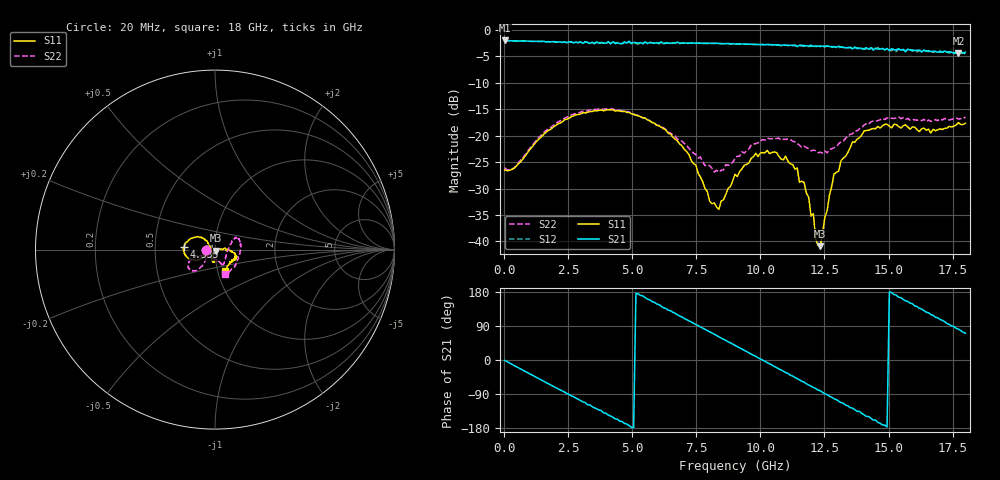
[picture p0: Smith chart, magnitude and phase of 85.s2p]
!Agilent Technologies,N5230A,US43500223,A.07.50.48
!Agilent N5230A: A.07.50.48
!Date: Monday, January 11, 2016 20:00:36
!Correction: S11(Full 2 Port(1,2))
!S21(Full 2 Port(1,2))
!S12(Full 2 Port(1,2))
!S22(Full 2 Port(1,2))
!S2P File: Measurements: S11, S21, S12, S22:
# Hz S  dB  R 50
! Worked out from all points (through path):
!   201 points, 20 MHz to 18 GHz, reference 50 ohm
!   highest |S21| = -1.97 dB at 20 MHz (marker M1); lowest = -4.3 dB at 17.73 GHz (marker M2)
!   group delay of S21, straight-line fit = 100 ps
!   lowest |S11| = -40.9 dB at 12.34 GHz (marker M3), VSWR 1.02, Z = 50.7 - j0.602 ohm
!   |S11| at or under -10 dB: start of sweep to end of sweep
!   |S22| runs from -26.9 to -14.8 dB; largest |S21 - S12| = 0.063
!   S11 on the Smith chart (normalised r, x): 20 MHz: 0.91, +0.00; 4.335 GHz: 0.71, +0.02; 18 GHz: 1.09, -0.26
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2e7  -26.48 179.6  -1.97 -0.8  -1.96 -0.9  -26.05 179.7
1.5483e9  -19.74 -146.9  -2.12 -56.2  -2.14 -56.8  -19.38 -129.0
3.0766e9  -15.63 -165.9  -2.52 -110.6  -2.45 -110.8  -15.36 -135.3
4.3352e9  -15.33 175.1  -2.58 -155.3  -2.44 -155.9  -15.13 -147.6
4.8746e9  -15.60 165.3  -2.10 -172.7  -2.22 -173.9  -15.46 -152.5
6.0433e9  -18.11 144.7  -2.48 146.0  -2.60 144.8  -18.05 -160.7
7.3918e9  -25.32 135.5  -2.44 97.0  -2.44 95.5  -23.30 -151.1
8.3807e9  -33.95 -150.0  -2.56 61.2  -2.56 59.5  -26.91 -108.3
9.01e9  -27.30 -100.5  -2.64 38.5  -2.66 36.4  -24.32 -78.7
1.00888e10  -23.19 -93.9  -2.74 -0.5  -2.71 -2.7  -20.71 -66.3
1.09878e10  -23.88 -108.7  -2.86 -33.1  -2.86 -35.4  -20.70 -58.0
1.1707e10  -28.85 -108.8  -2.92 -58.4  -3.03 -61.0  -22.00 -44.6
1.20666e10  -34.77 -96.3  -3.10 -72.4  -2.96 -74.6  -22.74 -30.2
1.21565e10  -39.56 -81.9  -3.00 -75.2  -3.11 -78.1  -22.84 -29.9
1.23363e10  -40.92 -41.4  -3.11 -81.0  -3.00 -84.3  -23.12 -20.9
1.28757e10  -27.25 -1.2  -3.13 -102.4  -3.12 -104.5  -22.28 5.0
1.31454e10  -24.74 7.6  -3.26 -112.4  -3.19 -114.2  -21.15 13.3
1.40444e10  -19.12 -9.5  -3.53 -144.5  -3.61 -146.7  -17.97 29.9
1.50333e10  -18.23 -20.3  -3.88 179.3  -3.90 176.3  -16.74 22.8
1.66515e10  -19.50 -39.0  -4.08 120.0  -3.92 116.3  -17.29 -25.1
1.77303e10  -17.53 -64.1  -4.35 81.3  -4.35 75.9  -16.86 -58.4
1.8e10  -17.65 -64.5  -4.19 70.7  -4.53 66.1  -16.46 -67.3
